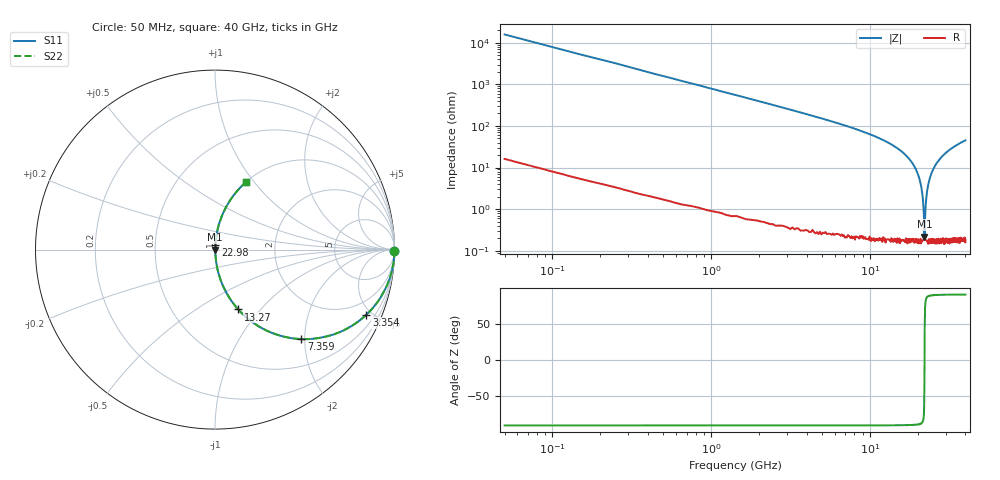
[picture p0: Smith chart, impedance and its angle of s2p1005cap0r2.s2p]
!	AVX	Thin	Film	Operation
!	Date:	March 2012
!	Description: Ultra-Miniature 01005 Size ACCU - P® Thin Film RF / Microwave Capacitor
!	Part Number:  C005YJ0R2ABSTR
!	Serial	Measurements
# MHZ S MA R 50
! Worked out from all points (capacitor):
!   400 points, 50 MHz to 40 GHz, reference 50 ohm
!   read as one part in series: C = 200 fF near 250.3 MHz
!   lowest |Z| = 219 mohm at 22.08 GHz (marker M1)
!   series resonance near 22.11 GHz, so ESL is about 260 pH
!   S11 on the Smith chart (normalised r, x): 50 MHz: open; 3.354 GHz: 1.00, -4.64; 7.359 GHz: 1.01, -1.92; 13.27 GHz: 1.00, -0.77; 22.98 GHz: 1.00, +0.06; 40 GHz: 1.00, +0.90
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50  1 -0.4  0.006283 89.6  0.006283 89.6  1 -0.4
150.125  1 -1.1  0.019 88.9  0.019 88.9  1 -1.1
250.251  0.999 -1.8  0.031 88.1  0.031 88.1  0.999 -1.8
750.877  0.995 -5.4  0.094 84.5  0.094 84.5  0.995 -5.4
1752.13  0.976 -12.5  0.216 77.4  0.216 77.4  0.976 -12.5
3354.135  0.918 -23.3  0.396 66.6  0.396 66.6  0.918 -23.3
6758.396  0.729 -43.1  0.683 46.8  0.683 46.8  0.729 -43.1
7359.148  0.692 -46.1  0.72 43.8  0.72 43.8  0.692 -46.1
13266.54  0.358 -68.8  0.932 21.0  0.932 21.0  0.358 -68.8
13366.67  0.353 -69.1  0.934 20.7  0.934 20.7  0.353 -69.1
17271.55  0.177 -79.3  0.983 10.2  0.983 10.2  0.177 -79.3
20075.06  0.069 -84.6  0.996 4.0  0.996 4.0  0.069 -84.6
21076.32  0.035 -85.2  0.998 2.0  0.998 2.0  0.035 -85.2
21576.94  0.018 -83.5  0.998 1.0  0.998 1.0  0.018 -83.5
21877.32  0.007896 -77.1  0.998 0.4  0.998 0.4  0.007896 -77.1
22077.57  0.002058 -34.4  0.998 0.1  0.998 0.1  0.002058 -34.4
22478.07  0.012 81.1  0.998 -0.7  0.998 -0.7  0.012 81.1
22978.7  0.028 84.9  0.998 -1.6  0.998 -1.6  0.028 84.9
24480.58  0.073 84.5  0.996 -4.2  0.996 -4.2  0.073 84.5
26783.46  0.137 81.4  0.989 -7.9  0.989 -7.9  0.137 81.4
33391.73  0.291 72.7  0.955 -16.9  0.955 -16.9  0.291 72.7
40000  0.411 65.5  0.91 -24.3  0.91 -24.3  0.411 65.5
